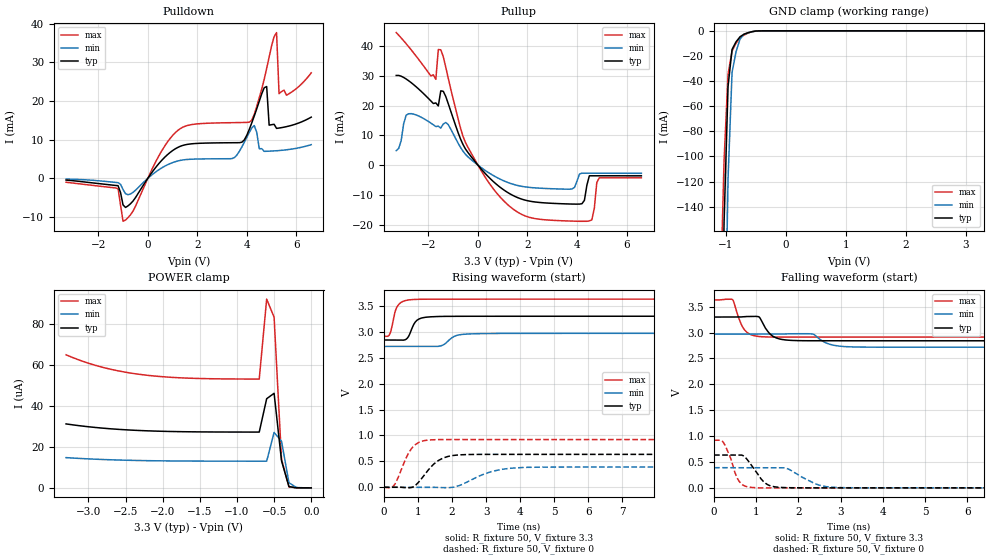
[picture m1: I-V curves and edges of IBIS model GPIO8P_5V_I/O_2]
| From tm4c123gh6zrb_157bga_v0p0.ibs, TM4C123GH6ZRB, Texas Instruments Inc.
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|   Model Cell GPIO8P_5V_I/O_2
[Model]   GPIO8P_5V_I/O_2
Model_type   I/O
Polarity   Non-Inverting
Enable   Active-Low
Vinl =  0.8
Vinh =  2
Cref =  15.0000pF
Rref =  100.0000M
Vref =  0V
Vmeas =  1.65
C_comp   4.711578p   4.034737p   5.423069p
[Model Spec]
Vinl   0.8   0.8   0.8
Vinh   2   2   2
[Temperature Range]   25   125   -40
[Voltage Range]   3.3   2.97   3.63
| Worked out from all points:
|   slope of the pulldown table from 0 to 0.495 V, typ, clamps not added: 118 ohm
|   slope of the pullup table from 0 to 0.495 V, typ, clamps not added: 109 ohm
|   GND clamp passes 1 mA (typ) near -0.59 V on its own axis
|   rising waveform, R_fixture 50, V_fixture 3.3: 20-80 % time 209ps typ, 304ps min, 170ps max; typ from 2.84 V to 3.3 V
|   rising waveform, R_fixture 50, V_fixture 0: 20-80 % time 527ps typ, 844ps min, 384ps max; typ from 0 V to 0.634 V
|   falling waveform, R_fixture 50, V_fixture 3.3: 20-80 % time 252ps typ, 337ps min, 213ps max; typ from 3.3 V to 2.84 V
|   falling waveform, R_fixture 50, V_fixture 0: 20-80 % time 342ps typ, 530ps min, 243ps max; typ from 0.634 V to 0 V
| Nom Voltages:
|   VDDC=1.2, VDD=3.3, GND=0
| Min Voltages:
|   VDDC=1.08, VDD=2.97, GND=0
| Max Voltages:
|   VDDC=1.32, VDD=3.63, GND=0
[POWER_clamp]
|   voltage   I(typ)   I(min)   I(max)
-3.3V     31.22uA    14.76uA    64.95uA
-3.1V     30.25uA    14.33uA    62.09uA
-2.8V     29.13uA    13.84uA    58.77uA
-2.3V     27.98uA    13.34uA    55.36uA
-1.7V     27.4uA     13.1uA     53.62uA
-700mV    27.24uA    13.03uA    53.12uA
-600mV    43.52uA    13.03uA    92.14uA
-500mV    46.16uA    27.05uA    83.3uA
-400mV    13.21uA    22.74uA    13.98uA
-300mV    630.7nA    2.501uA    480.9nA
-200mV    23.21nA    190.8nA    10.65nA
0V        660.4pA    10.19nA    564.9pA
[Pulldown]
|   voltage   I(typ)   I(min)   I(max)
-3.3V     -450.7uA   -192.2uA   -1.006mA
-1.2V     -1.893mA   -1.109mA   -2.697mA
-1V       -6.866mA   -2.892mA   -11.1mA
1.2V      7.958mA    4.478mA    12.33mA
3.5V      9.211mA    5.381mA    14.4mA
4.2V      14.36mA    13.04mA    15.06mA
4.5V      19.92mA    7.668mA    20.83mA
4.8V      23.73mA    7.004mA    28.42mA
4.9V      13.75mA    7.03mA     31.35mA
5.2V      12.91mA    7.14mA     37.68mA
5.3V      13mA       7.19mA     21.9mA
6.6V      15.82mA    8.714mA    27.27mA
[Pullup]
|   voltage   I(typ)   I(min)   I(max)
-3.3V     30.16mA    4.863mA    44.59mA
-2.9V     28.98mA    16.78mA    40.86mA
-1.7V     20.92mA    12.98mA    28.86mA
-1.6V     19.91mA    13.09mA    38.88mA
-1.5V     24.98mA    12.47mA    38.79mA
-500mV    5.386mA    3.597mA    7.551mA
1.6V      -10.92mA   -6.844mA   -15.8mA
3.8V      -13.1mA    -8.018mA   -18.83mA
4.2V      -12.99mA   -2.721mA   -18.9mA
4.5V      -3.591mA   -2.724mA   -18.76mA
4.9V      -3.59mA    -2.729mA   -4.279mA
6.6V      -3.606mA   -2.757mA   -4.278mA
[GND_clamp]
|   voltage   I(typ)   I(min)   I(max)
-3.3V     -16.3A     -15.26A    -17.13A
-1.1V     -340.4mA   -570.5mA   -222.8mA
-1.033V   -152.7mA   -296.8mA   -103.3mA
-966.7mV  -44.18mA   -117.7mA   -34.4mA
-900mV    -14.77mA   -33.12mA   -16.14mA
-833.3mV  -8.752mA   -16.68mA   -9.833mA
-766.7mV  -4.716mA   -6.551mA   -5.563mA
-700mV    -2.657mA   -2.741mA   -3.333mA
-566.7mV  -672.8uA   -727.2uA   -724.4uA
-433.3mV  -51.87uA   -90.8uA    -37.79uA
3.3V      660.4pA    5.308uA    422.7pA
[Ramp]
| variable   typ   min   max
dV/dt_f 0.28269897/0.25386606n 0.15654957/0.33829046n 0.43992818/0.21519855n
dV/dt_r 0.38699946/0.53401128n 0.23880101/0.85366195n 0.55927105/0.38819382n
R_load = 50
[Rising Waveform]
R_fixture = 50
V_fixture = 3.3
V_fixture_min = 2.97
V_fixture_max = 3.63
|   time   V(typ)   V(min)   V(max)
0s        2.841V     2.717V     2.912V
178.1ps   2.841V     2.717V     2.965V
341.5ps   2.841V     2.717V     3.419V
428.4ps   2.841V     2.717V     3.523V
687.2ps   2.877V     2.717V     3.61V
833.7ps   3.083V     2.717V     3.622V
1.166ns   3.274V     2.717V     3.628V
2.143ns   3.299V     2.931V     3.63V
2.818ns   3.299V     2.964V     3.63V
20.12ns   3.3V       2.97V      3.63V
[Rising Waveform]
R_fixture = 50
V_fixture = 0
V_fixture_min = 0
V_fixture_max = 0
|   time   V(typ)   V(min)   V(max)
0s        0V         0V         0V
320.1ps   0V         0V         57.85mV
634.7ps   -8.112mV   0V         543.5mV
833.3ps   0V         0V         764.8mV
1.337ns   360.6mV    0V         913.4mV
1.604ns   518.1mV    -4.493mV   919.6mV
2.025ns   613mV      0V         920.5mV
3.179ns   634.6mV    306.6mV    919.8mV
4.221ns   634.3mV    384.5mV    919.7mV
20.01ns   634.3mV    389.8mV    919.8mV
[Falling Waveform]
R_fixture = 50
V_fixture = 3.3
V_fixture_min = 2.97
V_fixture_max = 3.63
|   time   V(typ)   V(min)   V(max)
0s        3.3V       2.97V      3.63V
436.2ps   3.3V       2.97V      3.639V
720.2ps   3.308V     2.97V      3.054V
1.059ns   3.305V     2.97V      2.925V
1.179ns   3.141V     2.97V      2.917V
1.464ns   2.899V     2.97V      2.913V
2.039ns   2.843V     2.978V     2.913V
2.834ns   2.842V     2.755V     2.913V
3.318ns   2.841V     2.722V     2.913V
20.12ns   2.841V     2.717V     2.913V
[Falling Waveform]
R_fixture = 50
V_fixture = 0
V_fixture_min = 0
V_fixture_max = 0
|   time   V(typ)   V(min)   V(max)
0s        634.3mV    389.8mV    919.8mV
229.2ps   634.3mV    389.8mV    866.6mV
521.5ps   634.1mV    389.8mV    237.1mV
636.8ps   634.8mV    389.8mV    84.64mV
1.041ns   261.6mV    389.8mV    0V
1.409ns   23.56mV    389.7mV    0V
1.746ns   3.625mV    368.6mV    0V
2.48ns    0V         56.31mV    0V
3.006ns   0V         5.108mV    0V
20.01ns   0V         0V         0V
